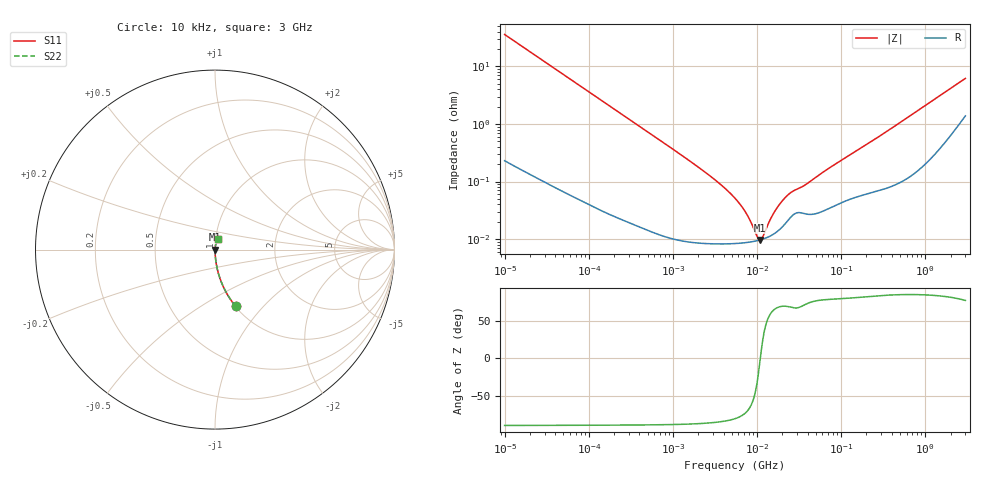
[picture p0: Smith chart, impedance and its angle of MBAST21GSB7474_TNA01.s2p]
! MBAST21GSB7474_TNA01  S-PARAMETER MODEL  ( Standard Model )
! Model Generated by TAIYO YUDEN Corporation (http://www.ty-top.com)
! Version 1.0
! TAIYO YUDEN Control No. 220601
! Copyright(c) 2012 TAIYO YUDEN CO.,LTD. All Rights Reserved.
! Product Description (link to TY-COMPAS)
! https://ds.yuden.co.jp/TYCOMPAS/or/detail?pn=MBAST21GSB7474KTNA01&u=M
! Products Name : Multilayer Ceramic Capacitors
! Characteristics :
!  Capacitance : 0.47 [uF] , Rated Voltage : 25 [V] , TCC : X7R
!  Case Size : 2.0 x 1.25 / 0.079 x 0.049 [mm/inch] , Thickness : 1.25 / 0.049 [mm/inch]
!  (Conditions: Temperature = 25 [degC] , DC Bias Voltage = 0 [V])
! External Node Assignments :
!  1  o---| |---o  2
! GND o---------o GND
! Frequency Range : 10kHz  -  3GHz  [ 401 STEP ]
# MHZ S RI R 50
! Freq[MHz].  S11 Real  S11 Imag  S21 Real  S21 Imag  S12 Real  S12 Imag  S22 Real  S22 Imag
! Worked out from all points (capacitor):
!   401 points, 10 kHz to 3 GHz, reference 50 ohm
!   read as one part in series: C = 443 nF near 10.65 kHz
!   lowest |Z| = 9.7 mohm at 10.96 MHz (marker M1)
!   series resonance near 10.95 MHz, so ESL is about 480 pH
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0.01  0.1156 -0.3165  0.8844 0.3165  0.8844 0.3165  0.1156 -0.3165
0.015549  0.0521 -0.2187  0.9479 0.2187  0.9479 0.2187  0.0521 -0.2187
0.026575  0.019 -0.1328  0.981 0.1328  0.981 0.1328  0.019 -0.1328
0.082683  0.00237 -0.0437  0.9976 0.0437  0.9976 0.0437  0.00237 -0.0437
0.683653  0.000148 -0.00535  0.9999 0.00535  0.9999 0.00535  0.000148 -0.00535
2.737278  8.47e-05 -0.00126  0.9999 0.00126  0.9999 0.00126  8.47e-05 -0.00126
4.124064  8.31e-05 -0.000768  0.9999 0.000768  0.9999 0.000768  8.31e-05 -0.000768
5.477226  8.4e-05 -0.000506  0.9999 0.000506  0.9999 0.000506  8.4e-05 -0.000506
7.274378  8.67e-05 -0.000284  0.9999 0.000284  0.9999 0.000284  8.67e-05 -0.000284
8.252149  8.88e-05 -0.000194  0.9999 0.000194  0.9999 0.000194  8.88e-05 -0.000194
9.97066  9.36e-05 -6.38e-05  0.9999 6.38e-05  0.9999 6.38e-05  9.36e-05 -6.38e-05
10.95979  9.7e-05 3.86e-07  0.9999 -3.86e-07  0.9999 -3.86e-07  9.7e-05 3.86e-07
12.04705  0.000101 6.47e-05  0.9999 -6.47e-05  0.9999 -6.47e-05  0.000101 6.47e-05
14.10408  0.000112 0.000174  0.9999 -0.000174  0.9999 -0.000174  0.000112 0.000174
15.99985  0.000124 0.000264  0.9999 -0.000264  0.9999 -0.000264  0.000124 0.000264
20.5901  0.000171 0.000455  0.9998 -0.000455  0.9998 -0.000455  0.000171 0.000455
25.67485  0.000247 0.000606  0.9998 -0.000606  0.9998 -0.000606  0.000247 0.000606
35.19136  0.000282 0.000777  0.9997 -0.000777  0.9997 -0.000777  0.000282 0.000777
45.28751  0.00027 0.00103  0.9997 -0.00103  0.9997 -0.00103  0.00027 0.00103
75.00035  0.000354 0.00174  0.9996 -0.00174  0.9996 -0.00174  0.000354 0.00174
374.4521  0.000857 0.0079  0.9991 -0.0079  0.9991 -0.0079  0.000857 0.0079
3000  0.0171 0.0584  0.9829 -0.0584  0.9829 -0.0584  0.0171 0.0584
